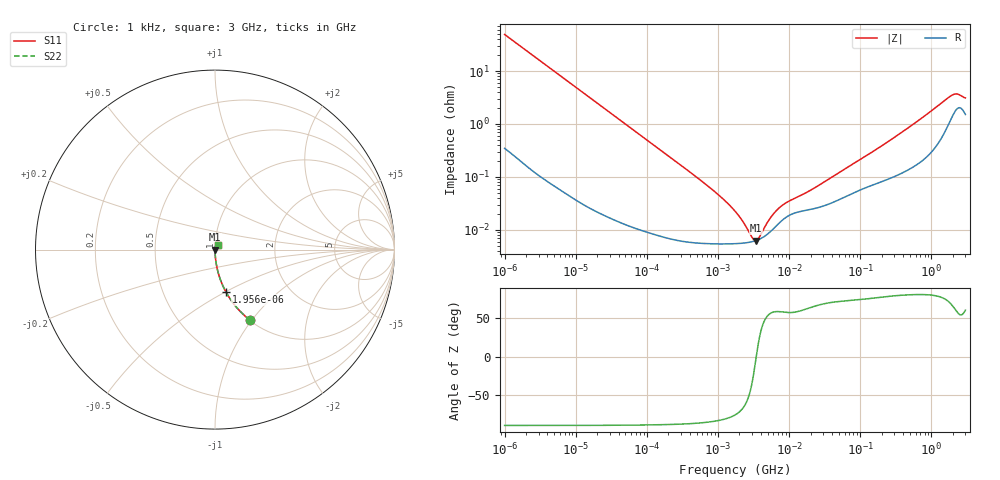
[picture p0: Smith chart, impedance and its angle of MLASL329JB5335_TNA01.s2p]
! MLASL329JB5335_TNA01  S-PARAMETER MODEL  ( Standard Model )
! Model Generated by TAIYO YUDEN Corporation (http://www.ty-top.com)
! Version 1.0
! TAIYO YUDEN Control No. 220601
! Copyright(c) 2009 TAIYO YUDEN CO.,LTD. All Rights Reserved.
! Product Description (link to TY-COMPAS)
! https://ds.yuden.co.jp/TYCOMPAS/or/detail?pn=MLASL329JB5335KTNA01&u=M
! Products Name : Multilayer Ceramic Capacitors
! Characteristics :
!  Capacitance : 3.3 [uF] , Rated Voltage : 10 [V] , TCC : B / X5R
!  Case Size : 3.2 x 2.5 / 0.126 x 0.098 [mm/inch] , Thickness : 0.85 / 0.033 [mm/inch]
!  (Conditions: Temperature = 25 [degC] , DC Bias Voltage = 0 [V])
! External Node Assignments :
!  1  o---| |---o  2
! GND o---------o GND
! Frequency Range : 1kHz  -  3GHz  [ 401 STEP ]
# MHZ S RI R 50
! Freq[MHz].  S11 Real  S11 Imag  S21 Real  S21 Imag  S12 Real  S12 Imag  S22 Real  S22 Imag
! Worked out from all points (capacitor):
!   401 points, 1 kHz to 3 GHz, reference 50 ohm
!   read as one part in series: C = 3.24 uF near 1.077 kHz
!   lowest |Z| = 6.27 mohm at 3.389 MHz (marker M1)
!   series resonance near 3.444 MHz, so ESL is about 660 pH
!   S11 on the Smith chart (normalised r, x): 1 kHz: 1.01, -0.98; 1.956 kHz: 1.00, -0.50; 3 GHz: 1.03, +0.05
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0.001  0.1955 -0.3931  0.8045 0.3931  0.8045 0.3931  0.1955 -0.3931
0.001452  0.1044 -0.3024  0.8956 0.3024  0.8956 0.3024  0.1044 -0.3024
0.001956  0.0608 -0.2358  0.9392 0.2358  0.9392 0.2358  0.0608 -0.2358
0.004443  0.0129 -0.1095  0.9871 0.1095  0.9871 0.1095  0.0129 -0.1095
0.01216  0.00197 -0.0406  0.998 0.0406  0.998 0.0406  0.00197 -0.0406
0.147855  8.84e-05 -0.00338  0.9999 0.00338  0.9999 0.00338  8.84e-05 -0.00338
0.791611  5.5e-05 -0.000604  0.9999 0.000604  0.9999 0.000604  5.5e-05 -0.000604
1.238299  5.44e-05 -0.000356  0.9999 0.000356  0.9999 0.000356  5.44e-05 -0.000356
1.732051  5.48e-05 -0.00022  0.9999 0.00022  0.9999 0.00022  5.48e-05 -0.00022
2.610246  5.76e-05 -8.38e-05  0.9999 8.38e-05  0.9999 8.38e-05  5.76e-05 -8.38e-05
2.812335  5.86e-05 -6.1e-05  0.9999 6.1e-05  0.9999 6.1e-05  5.86e-05 -6.1e-05
3.388684  6.25e-05 -4.86e-06  0.9999 4.86e-06  0.9999 4.86e-06  6.25e-05 -4.86e-06
4.083148  6.97e-05 5.15e-05  0.9999 -5.15e-05  0.9999 -5.15e-05  6.97e-05 5.15e-05
4.399271  7.39e-05 7.44e-05  0.9999 -7.44e-05  0.9999 -7.44e-05  7.39e-05 7.44e-05
6.153411  0.000108 0.000177  0.9999 -0.000177  0.9999 -0.000177  0.000108 0.000177
8.291982  0.000158 0.000256  0.9998 -0.000256  0.9998 -0.000256  0.000158 0.000256
21.06097  0.000247 0.000528  0.9998 -0.000528  0.9998 -0.000528  0.000247 0.000528
256.0921  0.000947 0.00472  0.9991 -0.00472  0.9991 -0.00472  0.000947 0.00472
650.4536  0.0019 0.0114  0.9981 -0.0114  0.9981 -0.0114  0.0019 0.0114
1917.819  0.0138 0.0312  0.9862 -0.0312  0.9862 -0.0312  0.0138 0.0312
2310.849  0.0201 0.03  0.9799 -0.03  0.9799 -0.03  0.0201 0.03
3000  0.0156 0.0263  0.9844 -0.0263  0.9844 -0.0263  0.0156 0.0263
